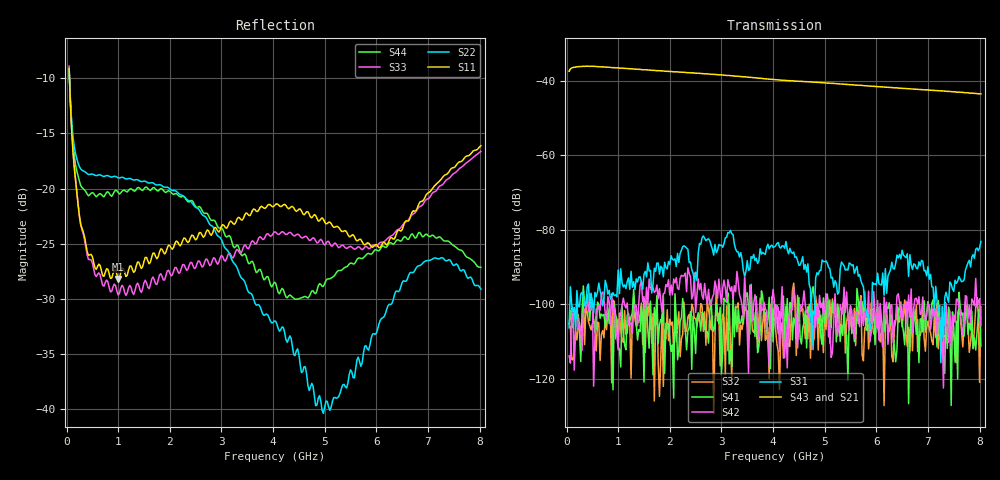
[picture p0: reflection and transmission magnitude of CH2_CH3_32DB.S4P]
!Agilent Technologies,E5071C,MY46316741,A.11.02
!Date: Thu May 28 14:41:21 2026
!Data & Calibration Information:
!1:CH2 INPUT 2:CH2 OUTPUT 3:CH3 INPUT 4:CH3 OUTPUT
!Freq	S11:SOLT4(ON)	S12:SOLT4(ON)	S13:SOLT4(ON)	S14:SOLT4(ON)
!	S21:SOLT4(ON)	S22:SOLT4(ON)	S23:SOLT4(ON)	S24:SOLT4(ON)
!	S31:SOLT4(ON)	S32:SOLT4(ON)	S33:SOLT4(ON)	S34:SOLT4(ON)
!	S41:SOLT4(ON)	S42:SOLT4(ON)	S43:SOLT4(ON)	S44:SOLT4(ON)
!PortZ  Port1:50+j0  Port2:50+j0  Port3:50+j0  Port4:50+j0
!Above PortZ is port z conversion or system Z0 setting when saving the data.
!When reading, reference impedance value at option line is always used.
# Hz S dB R 50
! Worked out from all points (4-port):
!   320 points, 50 MHz to 8.025 GHz, reference 50 ohm
!   strongest paths, dB at 50 MHz, 2.05 GHz, 4.05 GHz, 6.05 GHz, 8.025 GHz:
!     S43: -37.4, -37.5, -39.7, -41.6, -43.5
!     S21: -37.5, -37.6, -39.8, -41.8, -43.7
!     S31: -106.3, -87.9, -84.3, -94.5, -83.1
!     S42: -113.9, -97.4, -106.6, -109.6, -105.7
!     S41: -105.3, -110.9, -100.1, -104.1, -111.2
!     S32: -105.2, -104.7, -106.8, -107.8, -100.6
!   lowest |S11| = -28.2 dB at 1 GHz (marker M1), VSWR 1.08, Z = 47.7 - j3 ohm
!   |S11| at or under -10 dB: 57.11 MHz to end of sweep
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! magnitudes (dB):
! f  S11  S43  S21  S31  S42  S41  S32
! 50 MHz  -9.1  -37.4  -37.5  -106.3  -113.9  -105.3  -105.2
! 275 MHz  -23.3  -36.2  -36.2  -97.2  -106.7  -115.3  -113.3
! 1 GHz  -28.2  -36.5  -36.6  -90.8  -112.2  -111.4  -109.5
! 2.7 GHz  -24.0  -38.1  -38.2  -82.9  -97.7  -107.3  -111.0
! 4.975 GHz  -22.8  -40.5  -40.7  -88.5  -103.2  -98.3  -113.0
! 6.8 GHz  -21.7  -42.3  -42.5  -90.5  -100.0  -104.1  -112.7
! 8.025 GHz  -16.1  -43.5  -43.7  -83.1  -105.7  -111.2  -100.6
